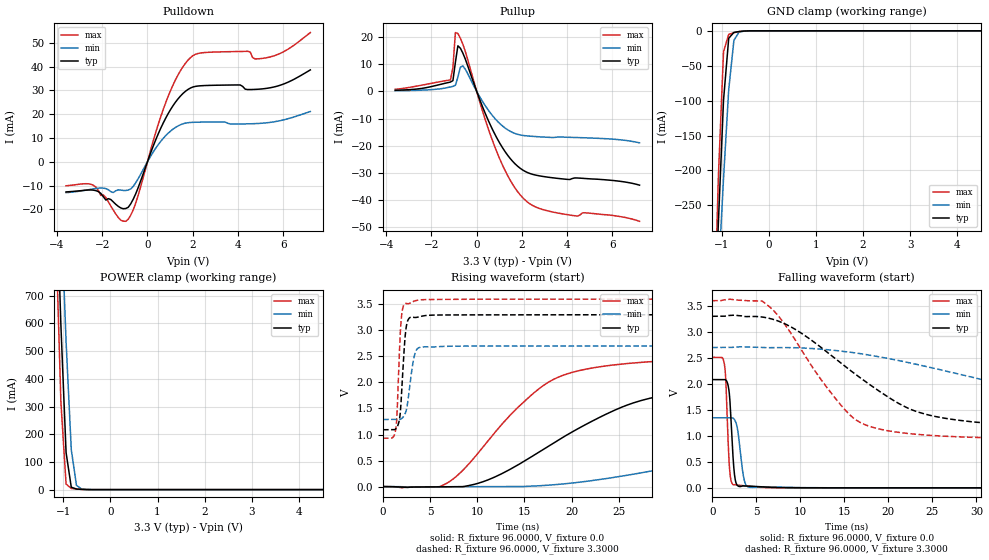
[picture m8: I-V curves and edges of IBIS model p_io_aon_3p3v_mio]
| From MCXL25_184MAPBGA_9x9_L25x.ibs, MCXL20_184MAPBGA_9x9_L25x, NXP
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[Model] p_io_aon_3p3v_mio
|   Model p_io_aon_3p3v_mio
| This model was characterised for following simulation conditions:
| External (pad) voltage:
|   - Typ: 3.3V,   - Min: 2.7V,   - Max: 3.6V
| Library cells for typ/min/max conditions are connected as defined below:
|  pad - External Pad
|  ipp_do_lv - Core Input
|  ipp_obe_lv - Output Buffer Enable
|  IOGC - NC
|  REFH3V3 - REFH3V3
|  REFL3V3 - REFL3V3
|  ZI - NC
|  abut_ncal_vddio[1] - vddio
|  abut_ncal_vddio[2] - vddio
|  abut_ncal_vddio[3] - vssio
|  abut_ncal_vddio[4] - vddio
|  abut_ncal_vddio[5] - vddio
|  abut_ncal_vddio[6] - vssio
|  abut_pcal_vddio[1] - vssio
|  abut_pcal_vddio[2] - vssio
|  abut_pcal_vddio[3] - vddio
|  abut_pcal_vddio[4] - vssio
|  abut_pcal_vddio[5] - vssio
|  abut_pcal_vddio[6] - vddio
|  ipp_do_1p8v - ipp_do_1p8v
|  ipp_eftd_lv - NC
|  ipp_ina_mux_vddio - NC
|  ipp_ina_mux_vddio[0] - NC
|  ipp_ina_mux_vddio[1] - NC
|  ipp_ina_r0_vddio - NC
|  ipp_ina_r0a_vddio - NC
|  ipp_ina_r0b_vddio - NC
|  ipp_ina_r0c_vddio - NC
|  ipp_ina_r0d_vddio - NC
|  ipp_ina_r0e_vddio - NC
|  ipp_ina_r0f_vddio - NC
|  ipp_ina_r300_vddio - NC
|  ipp_ina_r300a_vddio - NC
|  ipp_ina_r300b_vddio - NC
|  ipp_ina_r300c_vddio - NC
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Model_type I/O
Polarity   Non-Inverting
Enable   Active-High
Vinl =   0.9900V
Vinh =   2.3100V
Vmeas =  1.6500V
Cref =   30.0000pF
Rref =   1.0000M
Vref =   3.3000V
C_comp   1.3415pF   1.2957pF   1.4092pF
|C_comp_pullup   0.5415pF   0.5708pF   0.5218pF
|C_comp_pulldown   0.7031pF   0.7437pF   0.6731pF
[Model Spec]
| variable   typ   min   max
Vinh   2.3100V   1.8900V   2.5200V
Vinl   0.9900V   0.8100V   1.0800V
[Temperature Range]   25.0000   0.1250k   -40.0000
[Voltage Range]   3.3000V   2.7000V   3.6000V
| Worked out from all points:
|   slope of the pulldown table from 0 to 0.495 V, typ, clamps not added: 40.8 ohm
|   slope of the pullup table from 0 to 0.495 V, typ, clamps not added: 47.8 ohm
|   GND clamp passes 1 mA (typ) near -0.63 V on its own axis
|   POWER clamp passes 1 mA (typ) near -0.62 V on its own axis
|   rising waveform, R_fixture 96.0000, V_fixture 0.0: 20-80 % time 13.3ns typ, 27.8ns min, 8.16ns max; typ from 0 V to 2.08 V
|   rising waveform, R_fixture 96.0000, V_fixture 3.3000: 20-80 % time 452ps typ, 630ps min, 369ps max; typ from 1.09 V to 3.3 V
|   falling waveform, R_fixture 96.0000, V_fixture 0.0: 20-80 % time 424ps typ, 578ps min, 358ps max; typ from 2.08 V to 0 V
|   falling waveform, R_fixture 96.0000, V_fixture 3.3000: 20-80 % time 11.1ns typ, 24.1ns min, 6.71ns max; typ from 3.3 V to 1.09 V
[Pulldown]
|Voltage   I(typ)   I(min)   I(max)
-3.6V     -12.69mA   -13mA      -10.11mA
-2.39V    -11.94mA   -11.39mA   -9.907mA
-1.29V    -18.76mA   -11.81mA   -23.45mA
-960mV    -19.66mA   -12.1mA    -25.04mA
-520mV    -13.49mA   -8.854mA   -17.41mA
800mV     18.21mA    10.89mA    24.66mA
1.35V     26.41mA    15.03mA    36.46mA
1.79V     30.37mA    16.39mA    42.68mA
3V        32.13mA    16.71mA    46.1mA
4.43V     30.33mA    15.91mA    46.4mA
5.31V     30.89mA    16.4mA     43.78mA
7.2V      38.58mA    21.1mA     54.27mA
[Pullup]
|Voltage   I(typ)   I(min)   I(max)
-3.6V     377.7uA    207.8uA    734.8uA
-1.16V    3.397mA    1.602mA    4.185mA
-1.05V    3.926mA    1.816mA    8.675mA
-940mV    10.64mA    2.207mA    21.58mA
-830mV    16.7mA     5.22mA     21.24mA
-720mV    15.83mA    8.86mA     19.49mA
-610mV    14.01mA    9.302mA    17.31mA
820mV     -16.02mA   -10.13mA   -20.77mA
1.48V     -24.67mA   -14.68mA   -32.64mA
2.03V     -28.89mA   -16.19mA   -39.05mA
3.46V     -31.88mA   -16.93mA   -44.52mA
7.2V      -34.49mA   -18.94mA   -47.77mA
[GND_clamp]
|Voltage   I(typ)   I(min)   I(max)
-3.6V     -5.607A    -4.475A    -7.131A
-1.18V    -473.1mA   -501.9mA   -466.9mA
-1.07V    -276.4mA   -353.7mA   -210.9mA
-960mV    -99.46mA   -211.8mA   -30.01mA
-850mV    -10.76mA   -84.44mA   -5.071mA
-740mV    -2.289mA   -13.69mA   -2.754mA
-630mV    -1.015mA   -1.69mA    -1.169mA
-520mV    -313.8uA   -442.2uA   -284uA
7.2V      0A         0A         0A
[POWER_clamp]
|Voltage   I(typ)   I(min)   I(max)
-3.6V     14.37A     12.86A     16.2A
-1.16V    1.168A     1.525A     943.2mA
-1.05V    594.1mA    1.025A     315.9mA
-940mV    133.7mA    534mA      20.04mA
-830mV    8.718mA    144.9mA    4.268mA
-720mV    2.135mA    15.37mA    2.235mA
-610mV    851.7uA    1.853mA    843.3uA
7.2V      0A         0A         0A
[Ramp]
| variable   typ   min   max
dV/dt_r  1.2492/13.3318n   0.7994/27.7786n   1.5064/8.1551n
dV/dt_f  1.3248/11.0955n   0.8402/24.0792n   1.6025/6.7117n
R_load = 96.0000
[Rising Waveform]
R_fixture= 96.0000
V_fixture= 0.0
V_fixture_min= 0.0
V_fixture_max= 0.0
|time   V(typ)   V(min)   V(max)
0s        3.039nV    105.4nV    10.42nV
6.591ns   -4.422mV   -3.124mV   47.42mV
11.08ns   124.5mV    -1.781mV   864.7mV
17.03ns   717.9mV    20.73mV    1.943V
20.08ns   1.051V     68.39mV    2.194V
25.09ns   1.508V     193.8mV    2.349V
35.95ns   1.891V     553.2mV    2.459V
48.33ns   2.004V     935.5mV    2.494V
59.02ns   2.043V     1.114V     2.504V
128.4ns   2.082V     1.332V     2.511V
[Rising Waveform]
R_fixture= 96.0000
V_fixture= 3.3000
V_fixture_min= 2.7000
V_fixture_max= 3.6000
|time   V(typ)   V(min)   V(max)
0s        1.092V     1.289V     929.2mV
1.36ns    1.111V     1.289V     1.104V
1.497ns   1.146V     1.288V     1.442V
1.804ns   1.365V     1.29V      2.842V
2.113ns   2.254V     1.33V      3.442V
2.356ns   2.902V     1.405V     3.517V
2.582ns   3.165V     1.571V     3.513V
3.261ns   3.25V      2.463V     3.559V
3.831ns   3.26V      2.669V     3.584V
128.4ns   3.3V       2.7V       3.6V
[Falling Waveform]
R_fixture= 96.0000
V_fixture= 0.0
V_fixture_min= 0.0
V_fixture_max= 0.0
|time   V(typ)   V(min)   V(max)
0s        2.083V     1.349V     2.511V
1.38ns    2.084V     1.349V     2.382V
1.541ns   2.076V     1.349V     2.075V
1.958ns   1.79V      1.349V     395.6mV
2.145ns   1.271V     1.35V      137.3mV
2.43ns    437.5mV    1.333V     58.38mV
2.775ns   66.89mV    1.209V     54.68mV
3.649ns   36.19mV    141mV      40.68mV
4.366ns   32.36mV    10.36mV    26.86mV
128.4ns   561.5nV    7.96uV     45.43nV
[Falling Waveform]
R_fixture= 96.0000
V_fixture= 3.3000
V_fixture_min= 2.7000
V_fixture_max= 3.6000
|time   V(typ)   V(min)   V(max)
0s        3.3V       2.7V       3.6V
5.746ns   3.284V     2.698V     3.584V
7.619ns   3.201V     2.699V     3.285V
9.777ns   3.013V     2.693V     2.751V
15.77ns   2.247V     2.606V     1.381V
21.45ns   1.598V     2.439V     1.061V
30.33ns   1.257V     2.095V     967.7mV
41.64ns   1.156V     1.678V     940.2mV
52.02ns   1.123V     1.498V     933.3mV
128.4ns   1.092V     1.3V       929.2mV
